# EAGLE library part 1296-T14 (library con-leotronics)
1.27mm SINGLE ROW FEMALE SOCKET Source: http://www.leotronics.co.uk/Conexcon/Data%20Sheets/sec.%20A/1296ing.pdf
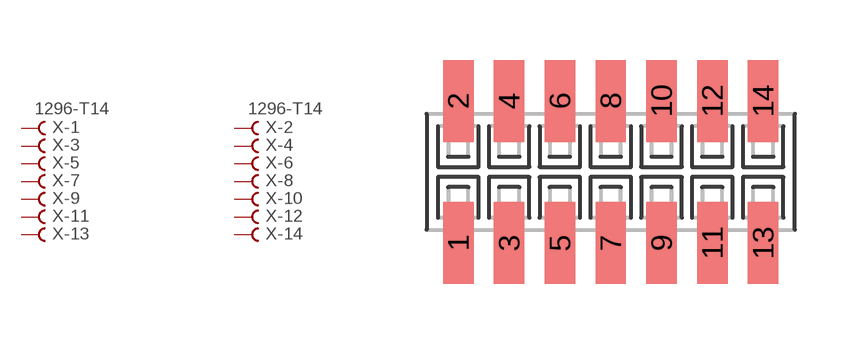
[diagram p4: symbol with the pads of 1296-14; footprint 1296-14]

Designator prefix X; gates -1=FVAL -2=FVAL -3=F -4=F -5=F -6=F -7=F -8=F -9=F -10=F -11=F -12=F -13=F -14=F

## 1296-T14 (OC_FARNELL: unknown; OC_NEWARK: unknown)  [1296-14]
1  -1:B  pas
2  -2:B  pas
3  -3:B  pas
4  -4:B  pas
5  -5:B  pas
6  -6:B  pas
7  -7:B  pas
8  -8:B  pas
9  -9:B  pas
10  -10:B  pas
11  -11:B  pas
12  -12:B  pas
13  -13:B  pas
14  -14:B  pas

## Footprint 1296-14 (pad centres in mm)
1.27mm SINGLE ROW FEMALE SOCKET Source: http://www.leotronics.co.uk/Conexcon/Data%20Sheets/sec.%20A/1296ing.pdf
smd 0.76 x 2.05: 1 -3.81,-1.78; 2 -3.81,1.78; 3 -2.54,-1.78; 4 -2.54,1.78; 5 -1.27,-1.78; 6 -1.27,1.78; 7 0,-1.78; 8 0,1.78; 9 1.27,-1.78; 10 1.27,1.78; 11 2.54,-1.78; 12 2.54,1.78; 13 3.81,-1.78; 14 3.81,1.78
